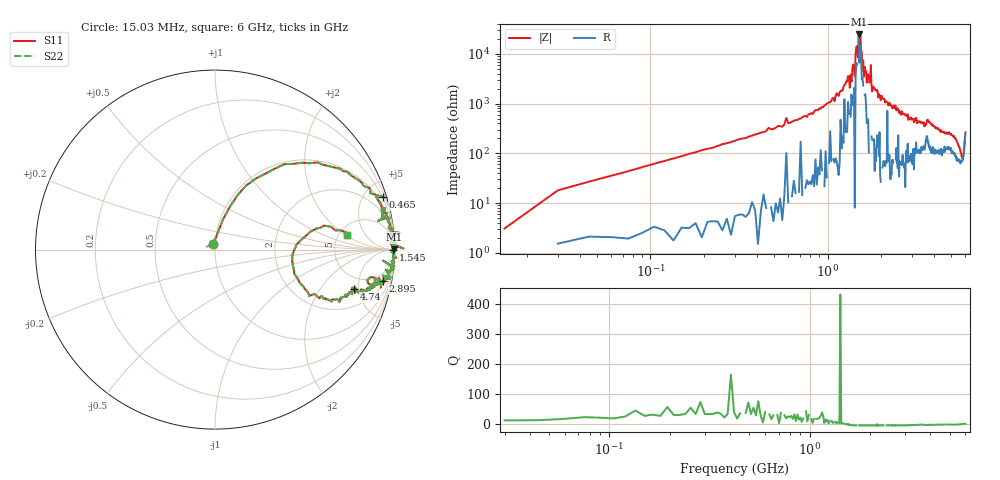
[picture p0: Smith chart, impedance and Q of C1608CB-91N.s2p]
!	Network	Analyzer	HP8753E.07.74:	Oct	30	2002	Serial	No.	JP38451487
!	Hewlett-Packard
!	28	Aug	2009	8:27:52
!	Frequency	S11	S21	S12	S22
#	HZ	S	RI	R	50
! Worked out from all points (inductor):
!   400 points, 15.03 MHz to 6 GHz, reference 50 ohm
!   read as one part in series: L = 94 nH near 45.03 MHz
!   highest |Z| = 24.7 kohm at 1.5 GHz (marker M1)
!   self-resonance near 1.5 GHz
!   S11 on the Smith chart (normalised r, x): 15.03 MHz: 0.98, +0.06; 465 MHz: 0.40, +6.52; 1.545 GHz: open; 2.895 GHz: 3, -10; 4.74 GHz: 3.57, -4.46; 6 GHz: 5.84, +2.15
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1.502992e7  -0.0101 0.0296  1.01 -0.0296  1.01 -0.0296  -0.0101 0.0296
3.002985e7  0.0449 0.169  0.955 -0.169  0.955 -0.169  0.0449 0.169
9.002955e7  0.229 0.397  0.771 -0.397  0.771 -0.397  0.229 0.397
4.650277e8  0.937 0.293  0.0633 -0.293  0.0633 -0.293  0.937 0.293
1.020025e9  0.986 0.0926  0.0144 -0.0926  0.0144 -0.0926  0.986 0.0926
1.425023e9  0.999 0.0286  0.000885 -0.0286  0.000885 -0.0286  0.999 0.0286
1.500022e9  0.996 0.000732  0.00397 -0.000732  0.00397 -0.000732  0.996 0.000732
1.515022e9  0.985 -0.000793  0.0146 0.000793  0.0146 0.000793  0.985 -0.000793
1.530022e9  0.997 -0.0033  0.0025 0.0033  0.0025 0.0033  0.997 -0.0033
1.545022e9  0.992 -9.16e-05  0.00778 9.16e-05  0.00778 9.16e-05  0.992 -9.16e-05
1.605022e9  1 -0.0281  -0.00463 0.0281  -0.00463 0.0281  1 -0.0281
1.725021e9  1 -0.0378  -0.00231 0.0378  -0.00231 0.0378  1 -0.0378
1.755021e9  1 0.0167  -6e-05 -0.0167  -6e-05 -0.0167  1 0.0167
1.785021e9  0.991 -0.0556  0.00909 0.0556  0.00909 0.0556  0.991 -0.0556
2.01002e9  0.995 -0.0712  0.00488 0.0712  0.00488 0.0712  0.995 -0.0712
2.895016e9  0.935 -0.174  0.0645 0.174  0.0645 0.174  0.935 -0.174
3.015015e9  0.941 -0.182  0.0588 0.182  0.0588 0.182  0.941 -0.182
4.00501e9  0.865 -0.224  0.135 0.224  0.135 0.224  0.865 -0.224
4.740006e9  0.776 -0.219  0.224 0.219  0.224 0.219  0.776 -0.219
5.010005e9  0.764 -0.235  0.236 0.235  0.236 0.235  0.764 -0.235
5.790001e9  0.43 -0.0622  0.57 0.0622  0.57 0.0622  0.43 -0.0622
6e9  0.734 0.0837  0.266 -0.0837  0.266 -0.0837  0.734 0.0837
